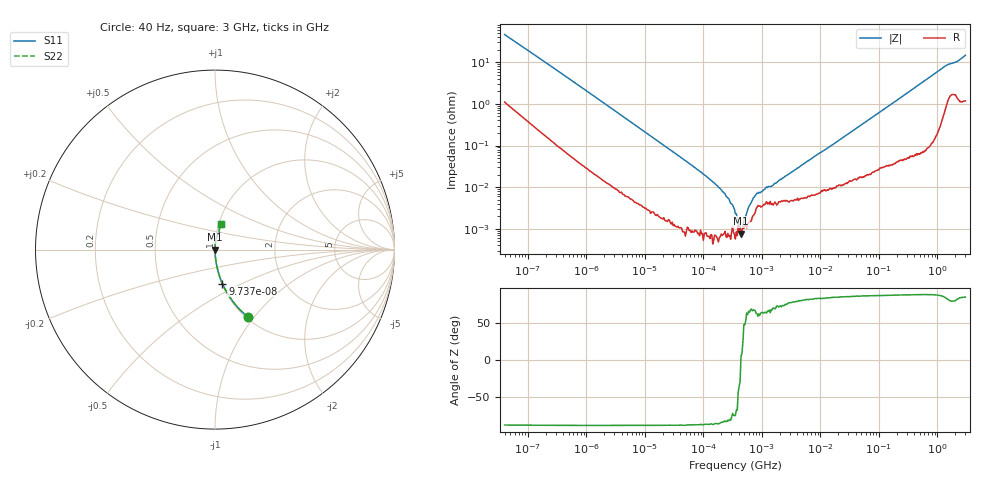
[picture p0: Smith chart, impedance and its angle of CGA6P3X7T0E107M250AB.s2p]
! S-Parameter Data Generated by TDK Corporation
! Copyright(C) 2024 TDK Corporation.
! All Rights Reserved.
! TDK P/N: CGA6P3X7T0E107M250AB (Multilayer Ceramic Chip Capacitor)
! Property: C=100uF
! Size(LxWxT): 0
! Model Type: s2p (Touchstone File Format Version 1.0)
! Frequency: DC=Yes Start=4E-05MHz Stop=3000MHz 622points Log-sweep
! Model Generated on May 28, 2024
! Terms and conditions regarding TDK Simulation Models:
! 1)This simulation model is being provided solely for informational
!  purposes. Please refer to the specifications of the products in
!  terms of detailed characteristics of such products.
! 2)In no event shall TDK Corporation of any of its subsidiaries be
!  liable for any loss or damage arising, directly or indirectly,
!  from any information contained in this simulation model, including,
!  but not limited to loss or damages arising from any inaccuracies,
!  omissions or errors in connection with such information.
! 3)Any and all copyrights on this simulation model are owned by
!  TDK Corporation.  Duplication or redistribution of this simulation
!  model without prior written permission from TDK Corporation
!  is prohibited.
! 4)This simulation model is subject to any modification or change
!  without any prior notice.
! 5)Neither TDK Corporation nor any of its subsidiaries shall make any
!  warranty, express or implied, including but not limited to the
!  correctness, implied warranties of merchantability and fitness for
!  a particular purpose with respect to this simulation models.
! 6)The use of this simulation model shall be deemed to have consented
!  to the terms and conditions hereof.
! Port Assignments:
!  1 ---| |--- 2
! Applicable Conditions:
!  Temperature = 25 degC
!  DC Bias Voltage = 0 V
!  Small Signal Operation
# Hz S MA R 50
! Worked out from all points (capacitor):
!   621 points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, 40 Hz to 3 GHz, reference 50 ohm
!   read as one part in series: C = 84.5 uF near 44.7 Hz
!   lowest |Z| = 768 uohm at 439.3 kHz (marker M1)
!   series resonance near 437.5 kHz, so ESL is about 1.6 nH
!   S11 on the Smith chart (normalised r, x): 40 Hz: 1.02, -0.93; 97.37 Hz: 1.01, -0.40; 3 GHz: 1.02, +0.30
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40  0.4195 -63.8  0.8978 24.8  0.8978 24.8  0.4195 -63.8
62.408  0.2894 -71.9  0.951 16.8  0.951 16.8  0.2894 -71.9
97.369  0.1943 -77.7  0.9771 11.2  0.9771 11.2  0.1943 -77.7
245.968  0.08105 -84.4  0.9954 4.6  0.9954 4.6  0.08105 -84.4
835.84  0.02467 -87.8  0.9994 1.4  0.9994 1.4  0.02467 -87.8
17465.72  0.001221 -89.0  1 0.1  1 0.1  0.001221 -89.0
82854.54  0.0002518 -88.2  1 0.0  1 0.0  0.0002518 -88.2
180460.1  9.861e-05 -87.2  1 0.0  1 0.0  9.861e-05 -87.2
201686.2  8.636e-05 -85.0  1 0.0  1 0.0  8.636e-05 -85.0
351682.9  2.298e-05 -75.7  1 0.0  1 0.0  2.298e-05 -75.7
439279.8  7.679e-06 5.1  1 -0.0  1 -0.0  7.679e-06 5.1
1109685  8.818e-05 64.7  1 -0.0  1 -0.0  8.818e-05 64.7
1386084  0.000104 64.2  1 -0.0  1 -0.0  0.000104 64.2
1607618  0.000118 70.0  1 -0.0  1 -0.0  0.000118 70.0
7348767  0.0005099 82.8  0.9999 -0.0  0.9999 -0.0  0.0005099 82.8
1.521322e7  0.0009857 84.6  0.9999 -0.1  0.9999 -0.1  0.0009857 84.6
1.49005e8  0.009095 87.4  0.9996 -0.5  0.9996 -0.5  0.009095 87.4
5.258324e8  0.03132 87.0  0.9988 -1.8  0.9988 -1.8  0.03132 87.0
1.320433e9  0.07839 80.9  0.9906 -4.5  0.9906 -4.5  0.07839 80.9
1.519029e9  0.08741 77.1  0.9842 -5.0  0.9842 -5.0  0.08741 77.1
2.134733e9  0.1017 76.2  0.9808 -5.8  0.9808 -5.8  0.1017 76.2
3e9  0.1448 77.1  0.978 -8.3  0.978 -8.3  0.1448 77.1
